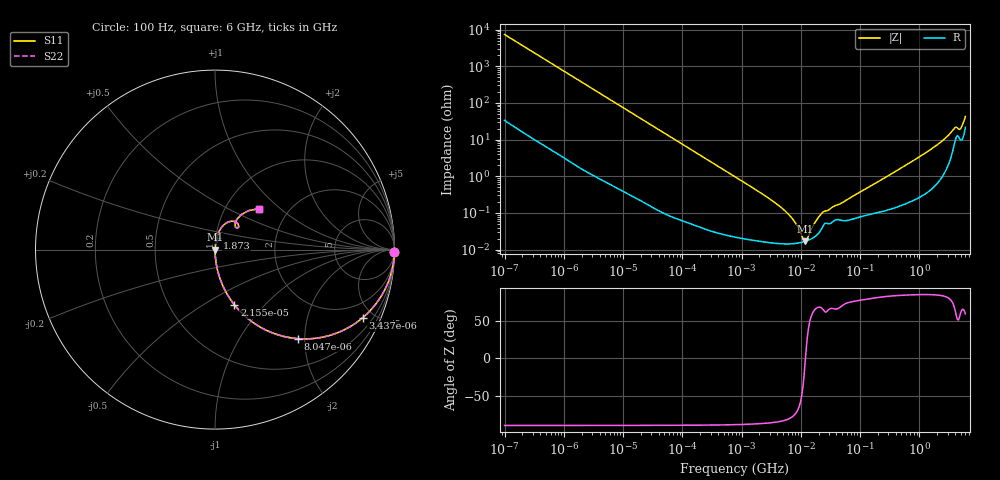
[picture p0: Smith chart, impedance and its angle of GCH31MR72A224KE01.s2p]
!Murata Part Number: GCH31MR72A224KE01
!These Parameters are Measured in Series Mode Connection
!Data Generated on Mar 13, 2026
!  o--ll--o
!Port1  Port2
!  o------o
!Operation Temp=25[degC], DC Bias Voltage=0[V]
!Freq. Start=100[Hz] Stop=6[GHz] 401[Steps]
# Hz S RI R 50
!Freq.(Hz) S11(Real) S11(Imag) S21(Real) S21(Imag) S12(Real) S12(Imag) S22(Real) S22(Imag)
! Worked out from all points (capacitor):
!   401 points, 100 Hz to 6 GHz, reference 50 ohm
!   read as one part in series: C = 216 nF near 109 Hz
!   lowest |Z| = 16.8 mohm at 11.89 MHz (marker M1)
!   series resonance near 11.97 MHz, so ESL is about 820 pH
!   S11 on the Smith chart (normalised r, x): 100 Hz: open; 3.437 kHz: 1.02, -4.31; 8.047 kHz: 1.01, -1.85; 21.55 kHz: 1.00, -0.69; 1.873 GHz: 1.01, +0.13; 6 GHz: 1.43, +0.74
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100  0.9998 -0.0136  0.000247 0.0136  0.000247 0.0136  0.9998 -0.0136
600  0.9931 -0.0807  0.0069 0.0807  0.0069 0.0807  0.9931 -0.0807
2008  0.9305 -0.2521  0.0695 0.2521  0.0695 0.2521  0.9305 -0.2521
3437  0.822 -0.3803  0.178 0.3803  0.178 0.3803  0.822 -0.3803
8047  0.4605 -0.4959  0.5395 0.4959  0.5395 0.4959  0.4605 -0.4959
21550  0.1083 -0.3079  0.8917 0.3079  0.8917 0.3079  0.1083 -0.3079
40335  0.0342 -0.1787  0.9658 0.1787  0.9658 0.1787  0.0342 -0.1787
129199  0.00388 -0.0578  0.9961 0.0578  0.9961 0.0578  0.00388 -0.0578
774597  0.000314 -0.00973  0.9997 0.00973  0.9997 0.00973  0.000314 -0.00973
5311619  0.000145 -0.00117  0.9999 0.00117  0.9999 0.00117  0.000145 -0.00117
7599586  0.000146 -0.000607  0.9999 0.000607  0.9999 0.000607  0.000146 -0.000607
1.087309e7  0.000161 -0.000125  0.9998 0.000125  0.9998 0.000125  0.000161 -0.000125
1.189169e7  0.000168 -8.7e-06  0.9998 8.7e-06  0.9998 8.7e-06  0.000168 -8.7e-06
1.300572e7  0.000177 0.000108  0.9998 -0.000108  0.9998 -0.000108  0.000177 0.000108
1.555665e7  0.000203 0.000347  0.9998 -0.000347  0.9998 -0.000347  0.000203 0.000347
1.946e7  0.000268 0.000673  0.9997 -0.000673  0.9997 -0.000673  0.000268 0.000673
2.434276e7  0.000472 0.000985  0.9995 -0.000985  0.9995 -0.000985  0.000472 0.000985
3.124326e8  0.00135 0.0107  0.9986 -0.0107  0.9986 -0.0107  0.00135 0.0107
1.873145e9  0.00989 0.0652  0.9901 -0.0652  0.9901 -0.0652  0.00989 0.0652
3.8344e9  0.0892 0.1582  0.9108 -0.1582  0.9108 -0.1582  0.0892 0.1582
5.016141e9  0.1116 0.1454  0.8884 -0.1454  0.8884 -0.1454  0.1116 0.1454
6e9  0.2475 0.2289  0.7525 -0.2289  0.7525 -0.2289  0.2475 0.2289
